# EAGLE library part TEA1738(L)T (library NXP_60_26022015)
GreenChip SMPS control IC The TEA1738GT is a low cost Switched Mode Power Supply (SMPS) controller IC intended for flyback topologies. It operates in peak current and frequency control mode. Frequency jitter has been implemented to reduce ElectroMagnetic Interference (EMI). Slope compensation is integrated for Continuous Conduction Mode (CCM) operation. The TEA1738GT IC includes OverPower Protection (OPP). This enables the controller to operate under overpower situations for a limited amount of time. Two pins, VINSENSE and PROTECT, are reserved for protection purposes. Input UnderVoltage Protection (UVP), output OverVoltage Protection (OVP) and OverTemperature Protection (OTP) can be implemented using a minimal number of external components. At low power levels the primary peak current is set to 25 % of the maximum peak current and the switching frequency is reduced to limit switching losses. The combination of fixed frequency operation at high output power and frequency reduction at low output power provides high efficiency over the total load range. The TEA1738GT enables low cost, highly efficient and reliable supplies for power requirements up to 75 W to be designed easily and with a minimum number of external components. The TEA1738GT is intended to operate in combination with a standby power supply. It has a lower start-up voltage than the TEA1738 AAL Eindhoven MK
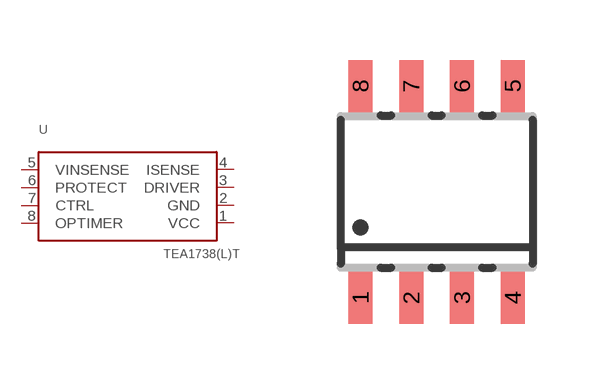
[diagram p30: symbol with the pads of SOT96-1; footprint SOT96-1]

Designator prefix U

## TEA1738(L)T (12NC: 9352 918 76118)  [SOT96-1]
1  VCC  pwr
2  GND  pwr
3  DRIVER  out
4  ISENSE  in
5  VINSENSE  in
6  PROTECT  in
7  CTRL  in
8  OPTIMER  pas

## Footprint SOT96-1 (pad centres in mm)
SOT96-1 SO8: plastic small outline package; 8 leads; body width 3.9 mm JEDEC: MS-012 IEC: 076E03
smd 0.6 x 1.3: 1 -1.905,-2.65; 2 -0.635,-2.65; 3 0.635,-2.65; 4 1.905,-2.65; 5 1.905,2.65; 6 0.635,2.65; 7 -0.635,2.65; 8 -1.905,2.65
